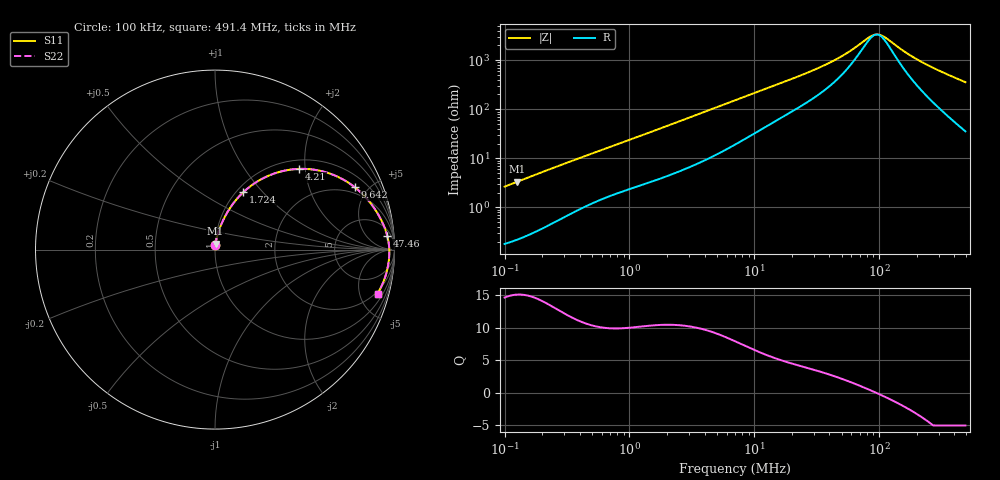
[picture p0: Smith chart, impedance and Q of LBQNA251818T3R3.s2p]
! LBQNA251818T3R3  S-PARAMETER MODEL  ( General Type )
! Model Generated by TAIYO YUDEN Corporation (http://www.ty-top.com)
! Version 1.0
! TAIYO YUDEN Control No. 191025NI43SB-FBB
! Copyright(c) 2019 TAIYO YUDEN CO.,LTD. All Rights Reserved.
! Product Description (link to TY-COMPAS)
! https://ds.yuden.co.jp/TYCOMPAS/or/detail?pn=LBQNA251818T3R3M&u=M
! Products Name : Inductors
! Characteristics :
!  Inductance : 3.3 uH , SRF(min) : 54 MHz , DC Resistance(max) : 0.143 Ohm
!  Rated Current : Saturation :440 mA , Temp Rise : 900 mA (20 degC)
!  Case Size : 2.5 x 1.8 / 0.098 x 0.071 [mm/inch] , Thickness : 1.8 / 0.071 [mm/inch]
!  (Conditions: Temperature = 25 degC , DC Bias Current/Voltage = 0A / 0V)
! External Node Assignments :
!  1  o---GGG---o  2
! GND o---------o GND
! Frequency Range : 0.1MHz  -  491.415554MHz  [ 402 STEP ]
# MHz S RI R 50
! Freq[MHz].  S11 Real  S11 Imag  S21 Real  S21 Imag  S12 Real  S12 Imag  S22 Real  S22 Imag
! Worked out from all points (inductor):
!   401 points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, 100 kHz to 491.4 MHz, reference 50 ohm
!   read as one part in series: L = 4.2 uH near 104.3 kHz
!   highest Q = 15.1 at 126.3 kHz (marker M1), where L = 4.2 uH
!   self-resonance near 95.44 MHz
!   S11 on the Smith chart (normalised r, x): 100 kHz: 1.00, +0.05; 1.724 MHz: 1.08, +0.79; 4.21 MHz: 1.19, +1.85; 9.642 MHz: 1.61, +4.09; 47.46 MHz: 10, +20; 491.4 MHz: 1.71, -7.09
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0.1  0.0025 0.0264  0.9975 -0.0264  0.9975 -0.0264  0.0025 0.0264
0.126332  0.0033 0.0332  0.9967 -0.0332  0.9967 -0.0332  0.0033 0.0332
0.415258  0.0201 0.1018  0.9799 -0.1018  0.9799 -0.1018  0.0201 0.1018
0.951117  0.0675 0.2058  0.9325 -0.2058  0.9325 -0.2058  0.0675 0.2058
1.72439  0.1584 0.3204  0.8416 -0.3204  0.8416 -0.3204  0.1584 0.3204
2.637593  0.28 0.4034  0.72 -0.4034  0.72 -0.4034  0.28 0.4034
4.209568  0.4682 0.4497  0.5318 -0.4497  0.5318 -0.4497  0.4682 0.4497
7.010104  0.6784 0.4085  0.3216 -0.4085  0.3216 -0.4085  0.6784 0.4085
9.641704  0.7783 0.3479  0.2217 -0.3479  0.2217 -0.3479  0.7783 0.3479
15.71854  0.8757 0.2468  0.1243 -0.2468  0.1243 -0.2468  0.8757 0.2468
29.11  0.9369 0.1418  0.0631 -0.1418  0.0631 -0.1418  0.9369 0.1418
47.45702  0.9597 0.0769  0.0403 -0.0769  0.0403 -0.0769  0.9597 0.0769
59.9536  0.9657 0.0498  0.0343 -0.0498  0.0343 -0.0498  0.9657 0.0498
82.46025  0.9701 0.0154  0.0299 -0.0154  0.0299 -0.0154  0.9701 0.0154
89.77577  0.9707 0.00644  0.0293 -0.00644  0.0293 -0.00644  0.9707 0.00644
95.68525  0.971 -0.000271  0.029 0.000271  0.029 0.000271  0.971 -0.000271
101.9837  0.9711 -0.00701  0.0289 0.00701  0.0289 0.00701  0.9711 -0.00701
120.8815  0.971 -0.0252  0.029 0.0252  0.029 0.0252  0.971 -0.0252
162.7648  0.9686 -0.0592  0.0314 0.0592  0.0314 0.0592  0.9686 -0.0592
219.16  0.9626 -0.098  0.0374 0.098  0.0374 0.098  0.9626 -0.098
328.1747  0.9447 -0.1629  0.0553 0.1629  0.0553 0.1629  0.9447 -0.1629
491.4156  0.906 -0.2461  0.094 0.2461  0.094 0.2461  0.906 -0.2461
